TYPE EC_SLAVE_DIAG_INFO_DATA :
STRUCT
	Addr									:	WORD; //Slaves own physical address e.g. 1004 
	ConfigType								:	STRING(18); //Configured type e.g. EL1008 or EL7211 
	ConfigName								:	STRING(31); //Name as configured in IO-tree (type removed)
	ConfigTypeIdentity						:	STRING(18); //Configured type according identity e.g. AX5206-0000-0210

	{attribute 'displaymode':='hex'}  
	DevState								:	BYTE; //Device state constant e.g. 16#08=Tc2_EtherCAT.EC_DEVICE_STATE_OP
	DevStateText							:	STRING(60) := 'Hello'; //e.g. OP, INIT etc...
	

	{attribute 'displaymode':='hex'}  
	LinkState								:	BYTE; //Link state constant e.g. 0=Tc2_EtherCAT.EC_LINK_STATE_NOT_PRESENT



	//Error information	
	CntOfCRCErrors							:	UDINT; //Total number of CRC-Errors on all four ports of the slave 

	ConfigIdentity							:	ST_EcSlaveIdentity; //EtherCAT identity data of an EtherCAT slave device, vendor Id, product code etc...

END_STRUCT
END_TYPE
